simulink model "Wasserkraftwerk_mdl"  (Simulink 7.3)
settings: Solver=ode23tb  StartTime=0.0  StopTime=1000  MaxStep=0.1  RelTol=1e-4
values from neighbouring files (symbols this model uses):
  A_V0 = 0.518    [Parameter_sim.m]
  A_W = 5^2*pi    (= 78.5398163397)    [Parameter_sim.m]
  c_d = 0.9658    [Parameter_sim.m]
  d_F = 2    [Parameter_sim.m]
  d_T = 3    [Parameter_sim.m]
  d_Turb = 5.35    [Parameter_sim.m]
  g = 9.81    [Parameter_sim.m]
  h_R = 413    [Parameter_sim.m]
  h_W0 = 390    [Parameter_sim.m]
  h_W_IC = 413    [Parameter_sim.m]
  I_IC = 0    [Parameter_sim.m]
  kappa = 8.7*10^3    (= 8700)    [Parameter_sim.m]
  l_F = 741    [Parameter_sim.m]
  L_net = 0.1    [Parameter_sim.m]
  l_T = 2000    [Parameter_sim.m]
  L_tot = L_G+L_net    (= 0.2)    [Parameter_sim.m]
  lambda_F = 0.0153    [Parameter_sim.m]
  lambda_T = 0.0182    [Parameter_sim.m]
  lambda_W = 4.0738    [Parameter_sim.m]
  omega_IC = 0    [Parameter_sim.m]
  p_0 = 0    [Parameter_sim.m]
  R_net = 165    [Parameter_sim.m]
  R_tot = R_G+R_net    (= 175)    [Parameter_sim.m]
  rho = 1000    [Parameter_sim.m]
  sigma_0 = 6.2790e-010    (= 6.279e-10)    [Parameter_sim.m]
  Theta = 5.4997*10^3    (= 5499.7)    [Parameter_sim.m]
  v_F_IC = 0    [Parameter_sim.m]
  V_F_IC = l_F*pi*d_F^2/4    (= 2327.92015631)    [Parameter_sim.m]
  v_T_IC = 0    [Parameter_sim.m]
  x_IC = 0    [Parameter_sim.m]
undefined symbols (not defined in the file or in its folder): sigbuilder_block

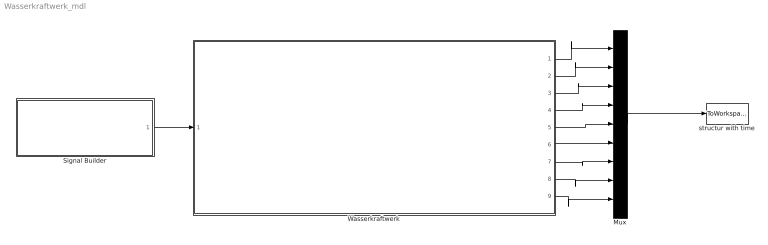
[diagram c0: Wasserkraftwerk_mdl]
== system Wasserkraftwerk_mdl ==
  Mux : Mux  Inputs=9
  Signal Builder : Subsystem  Tag=STV Subsys  LoadFcn=sigbuilder_block('load');  StartFcn=sigbuilder_block('start');  StopFcn=sigbuilder_block('stop');  ClipboardFcn=sigbuilder_block('clipboard');
  Wasserkraftwerk : Subsystem
  structur with time : ToWorkspace  VariableName=sim_daten  SampleTime=-1  SaveFormat=Structure With Time
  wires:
  Signal Builder/1(u) -> Wasserkraftwerk/1(u)
  Mux/1 -> structur with time/1
  Wasserkraftwerk/1(x) -> Mux/1
  Wasserkraftwerk/2(h_W) -> Mux/2
  Wasserkraftwerk/3(p_F) -> Mux/3
  Wasserkraftwerk/4(V_flw_T) -> Mux/4
  Wasserkraftwerk/5(V_flw_F) -> Mux/5
  Wasserkraftwerk/6(omega) -> Mux/6
  Wasserkraftwerk/7(U) -> Mux/7
  Wasserkraftwerk/8(I) -> Mux/8
  Wasserkraftwerk/9(P) -> Mux/9

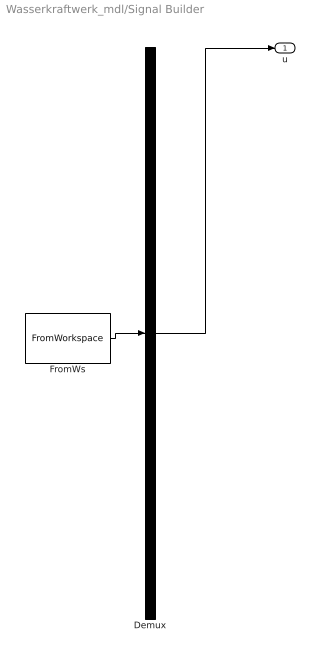
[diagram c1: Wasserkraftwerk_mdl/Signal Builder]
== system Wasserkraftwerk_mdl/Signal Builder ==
  Demux : Demux  Tag=STV Demux  Outputs=1
  FromWs : FromWorkspace  Tag=STV FromWs  VariableName=tuvar  SampleTime=0  SigBuilderData=DataTag0  VnvData=DataTag1
  u : Outport  Tag=STV Outport  OutDataType=sfix(16)  OutScaling=2^0
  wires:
  Demux/1 -> u/1
  FromWs/1 -> Demux/1

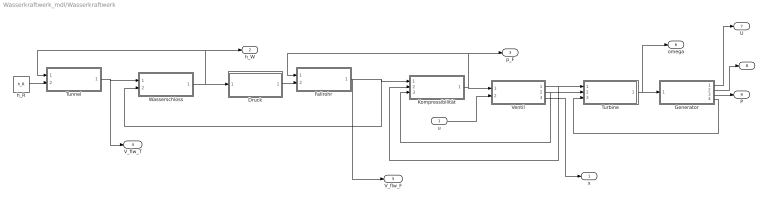
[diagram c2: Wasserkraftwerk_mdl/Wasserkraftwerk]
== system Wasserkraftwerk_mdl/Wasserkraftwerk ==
  u : Inport  OutDataType=sfix(16)  OutScaling=2^0
  Druck : Subsystem
  Fallrohr : Subsystem
  Generator : Subsystem
  Kompressibilität : Subsystem
  Tunnel : Subsystem
  Turbine : Subsystem
  Ventil : Subsystem
  Wasserschloss : Subsystem
  h_R : Constant  Value=h_R  OutDataType=sfix(16)  OutScaling=2^0
  x : Outport  OutDataType=sfix(16)  OutScaling=2^0
  h_W : Outport  Port=2  OutDataType=sfix(16)  OutScaling=2^0
  p_F : Outport  Port=3  OutDataType=sfix(16)  OutScaling=2^0
  V_flw_T : Outport  Port=4  OutDataType=sfix(16)  OutScaling=2^0
  V_flw_F : Outport  Port=5  OutDataType=sfix(16)  OutScaling=2^0
  omega : Outport  Port=6  OutDataType=sfix(16)  OutScaling=2^0
  U : Outport  Port=7  OutDataType=sfix(16)  OutScaling=2^0
  I : Outport  Port=8  OutDataType=sfix(16)  OutScaling=2^0
  P : Outport  Port=9  OutDataType=sfix(16)  OutScaling=2^0
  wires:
  Wasserschloss/1(h_W) -> Druck/1(h_W), Tunnel/1(h_W), h_W/1
  Kompressibilität/1(p_F) -> Ventil/1(p_F), Fallrohr/1(p_F), p_F/1
  Ventil/1(v_V) -> Kompressibilität/2(v_V), Turbine/1(v_V)
  Turbine/1(omega) -> Generator/1(omega), omega/1
  Ventil/2(A_V) -> Kompressibilität/3(A_V), Turbine/2(A_V)
  Generator/1(U) -> U/1
  Generator/2(I) -> I/1
  u/1 -> Ventil/2(u)
  Druck/1(p_W) -> Fallrohr/2(p_W)
  Generator/4(T_G) -> Turbine/3(T_G)
  Ventil/3(x) -> x/1
  Tunnel/1(V_flw_T) -> V_flw_T/1, Wasserschloss/1(V_flw_T)
  Fallrohr/1(V_flw_F) -> Kompressibilität/1(V_flw_F), Wasserschloss/2(V_flw_F), V_flw_F/1
  Generator/3(P) -> P/1
  h_R/1 -> Tunnel/2(h_R)

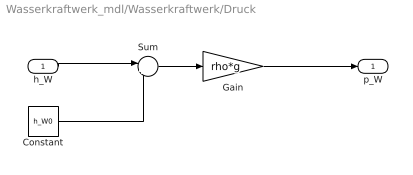
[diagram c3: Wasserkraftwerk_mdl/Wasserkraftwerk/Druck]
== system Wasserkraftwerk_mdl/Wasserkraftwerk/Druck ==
  h_W : Inport  OutDataType=sfix(16)  OutScaling=2^0
  Constant : Constant  Value=h_W0  OutDataType=sfix(16)  OutScaling=2^0
  Gain : Gain  Gain=rho*g  ParameterDataType=sfix(16)  ParameterScaling=2^0  OutDataType=sfix(16)  OutScaling=2^0
  Sum : Sum  Inputs=|+-  OutDataType=sfix(16)  OutScaling=2^0
  p_W : Outport  OutDataType=sfix(16)  OutScaling=2^0
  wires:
  h_W/1 -> Sum/1
  Constant/1 -> Sum/2
  Sum/1 -> Gain/1
  Gain/1 -> p_W/1

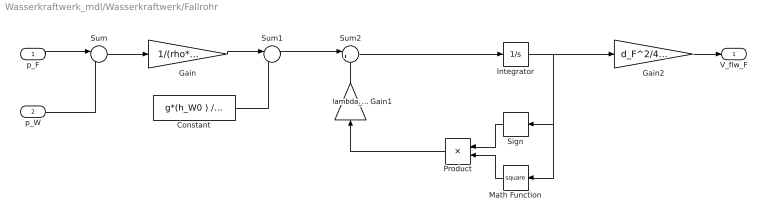
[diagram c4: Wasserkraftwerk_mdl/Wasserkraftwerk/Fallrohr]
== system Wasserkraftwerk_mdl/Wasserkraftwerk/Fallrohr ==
  p_F : Inport  OutDataType=sfix(16)  OutScaling=2^0
  p_W : Inport  Port=2  OutDataType=sfix(16)  OutScaling=2^0
  Constant : Constant  Value=g*(h_W0 ) / l_F  OutDataType=sfix(16)  OutScaling=2^0
  Gain : Gain  Gain=1/(rho*l_F)  ParameterDataType=sfix(16)  ParameterScaling=2^0  OutDataType=sfix(16)  OutScaling=2^0
  Gain1 : Gain  Gain=lambda_F/(2*d_F)  ParameterDataType=sfix(16)  ParameterScaling=2^0  OutDataType=sfix(16)  OutScaling=2^0
  Gain2 : Gain  Gain=d_F^2/4*pi  ParameterDataType=sfix(16)  ParameterScaling=2^0  OutDataType=sfix(16)  OutScaling=2^0
  Integrator : Integrator  InitialCondition=v_F_IC
  Math Function : Math  Operator=square  OutDataType=sfix(16)  OutScaling=2^0
  Product : Product  OutDataType=sfix(16)  OutScaling=2^0
  Sign : Signum
  Sum : Sum  Inputs=|-+  OutDataType=sfix(16)  OutScaling=2^0
  Sum1 : Sum  Inputs=|++  OutDataType=sfix(16)  OutScaling=2^0
  Sum2 : Sum  Inputs=|+-  OutDataType=sfix(16)  OutScaling=2^0
  V_flw_F : Outport  OutDataType=sfix(16)  OutScaling=2^0
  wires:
  p_F/1 -> Sum/1
  p_W/1 -> Sum/2
  Sum/1 -> Gain/1
  Gain/1 -> Sum1/1
  Constant/1 -> Sum1/2
  Sum1/1 -> Sum2/1
  Sum2/1 -> Integrator/1
  Sign/1 -> Product/1
  Math Function/1 -> Product/2
  Product/1 -> Gain1/1
  Gain1/1 -> Sum2/2
  Integrator/1 -> Sign/1, Math Function/1, Gain2/1
  Gain2/1 -> V_flw_F/1

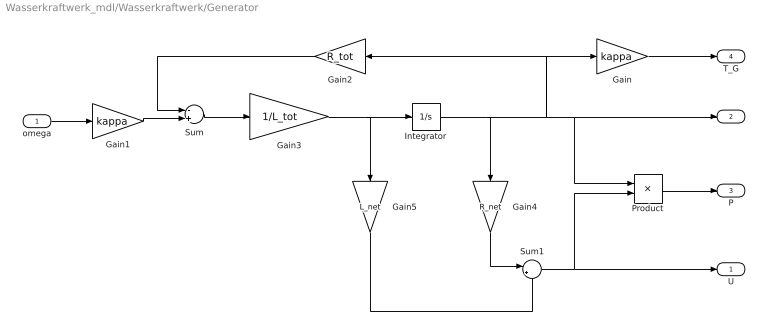
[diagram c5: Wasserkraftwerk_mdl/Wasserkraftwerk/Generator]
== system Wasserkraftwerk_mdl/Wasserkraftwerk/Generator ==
  omega : Inport  OutDataType=sfix(16)  OutScaling=2^0
  Gain : Gain  Gain=kappa  ParameterDataType=sfix(16)  ParameterScaling=2^0  OutDataType=sfix(16)  OutScaling=2^0
  Gain1 : Gain  Gain=kappa  ParameterDataType=sfix(16)  ParameterScaling=2^0  OutDataType=sfix(16)  OutScaling=2^0
  Gain2 : Gain  Gain=R_tot  ParameterDataType=sfix(16)  ParameterScaling=2^0  OutDataType=sfix(16)  OutScaling=2^0
  Gain3 : Gain  Gain=1/L_tot  ParameterDataType=sfix(16)  ParameterScaling=2^0  OutDataType=sfix(16)  OutScaling=2^0
  Gain4 : Gain  Gain=R_net  ParameterDataType=sfix(16)  ParameterScaling=2^0  OutDataType=sfix(16)  OutScaling=2^0
  Gain5 : Gain  Gain=L_net  ParameterDataType=sfix(16)  ParameterScaling=2^0  OutDataType=sfix(16)  OutScaling=2^0
  Integrator : Integrator  InitialCondition=I_IC
  Product : Product  OutDataType=sfix(16)  OutScaling=2^0
  Sum : Sum  Inputs=-+  OutDataType=sfix(16)  OutScaling=2^0
  Sum1 : Sum  Inputs=|++  OutDataType=sfix(16)  OutScaling=2^0
  U : Outport  OutDataType=sfix(16)  OutScaling=2^0
  I : Outport  Port=2  OutDataType=sfix(16)  OutScaling=2^0
  P : Outport  Port=3  OutDataType=sfix(16)  OutScaling=2^0
  T_G : Outport  Port=4  OutDataType=sfix(16)  OutScaling=2^0
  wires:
  Integrator/1 -> Gain/1, Gain2/1, I/1, Product/1, Gain4/1
  Gain/1 -> T_G/1
  omega/1 -> Gain1/1
  Gain2/1 -> Sum/1
  Gain1/1 -> Sum/2
  Sum/1 -> Gain3/1
  Gain3/1 -> Gain5/1, Integrator/1
  Sum1/1 -> U/1, Product/2
  Gain4/1 -> Sum1/1
  Gain5/1 -> Sum1/2
  Product/1 -> P/1

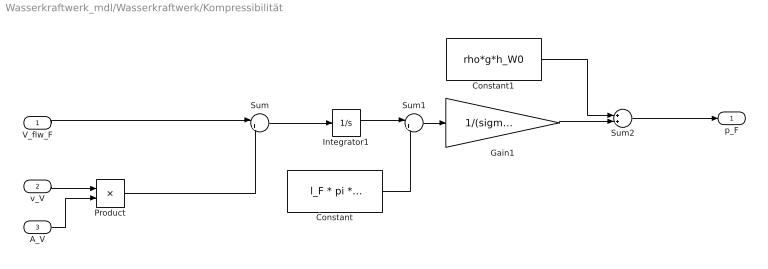
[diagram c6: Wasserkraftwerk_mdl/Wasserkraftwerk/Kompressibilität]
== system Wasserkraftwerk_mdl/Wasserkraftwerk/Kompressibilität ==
  V_flw_F : Inport  OutDataType=sfix(16)  OutScaling=2^0
  v_V : Inport  Port=2  OutDataType=sfix(16)  OutScaling=2^0
  A_V : Inport  Port=3  OutDataType=sfix(16)  OutScaling=2^0
  Constant : Constant  Value=l_F * pi * d_F^2 / 4  OutDataType=sfix(16)  OutScaling=2^0
  Constant1 : Constant  Value=rho*g*h_W0  OutDataType=sfix(16)  OutScaling=2^0
  Gain1 : Gain  Gain=1/(sigma_0 * l_F*pi*d_F^2/4)  ParameterDataType=sfix(16)  ParameterScaling=2^0  OutDataType=sfix(16)  OutScaling=2^0
  Integrator1 : Integrator  InitialCondition=V_F_IC
  Product : Product  OutDataType=sfix(16)  OutScaling=2^0
  Sum : Sum  Inputs=|+-  OutDataType=sfix(16)  OutScaling=2^0
  Sum1 : Sum  Inputs=|+-  OutDataType=sfix(16)  OutScaling=2^0
  Sum2 : Sum  OutDataType=sfix(16)  OutScaling=2^0
  p_F : Outport  OutDataType=sfix(16)  OutScaling=2^0
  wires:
  v_V/1 -> Product/1
  A_V/1 -> Product/2
  Product/1 -> Sum/2
  Sum/1 -> Integrator1/1
  Constant/1 -> Sum1/2
  Sum1/1 -> Gain1/1
  Integrator1/1 -> Sum1/1
  Gain1/1 -> Sum2/2
  Sum2/1 -> p_F/1
  Constant1/1 -> Sum2/1
  V_flw_F/1 -> Sum/1

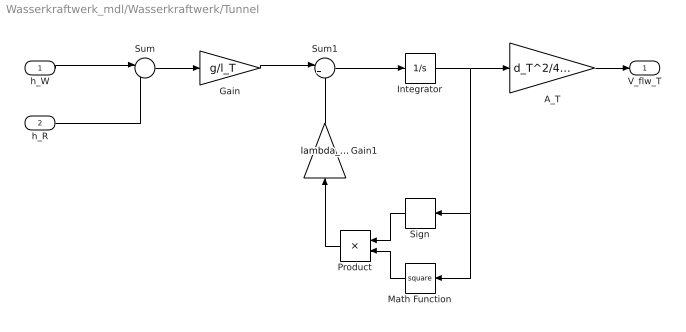
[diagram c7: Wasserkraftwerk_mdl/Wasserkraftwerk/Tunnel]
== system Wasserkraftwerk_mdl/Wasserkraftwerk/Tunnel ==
  h_W : Inport  OutDataType=sfix(16)  OutScaling=2^0
  h_R : Inport  Port=2  OutDataType=sfix(16)  OutScaling=2^0
  A_T : Gain  Gain=d_T^2/4*pi  ParameterDataType=sfix(16)  ParameterScaling=2^0  OutDataType=sfix(16)  OutScaling=2^0
  Gain : Gain  Gain=g/l_T  ParameterDataType=sfix(16)  ParameterScaling=2^0  OutDataType=sfix(16)  OutScaling=2^0
  Gain1 : Gain  Gain=lambda_T/(2*d_T)  ParameterDataType=sfix(16)  ParameterScaling=2^0  OutDataType=sfix(16)  OutScaling=2^0
  Integrator : Integrator  InitialCondition=v_T_IC
  Math Function : Math  Operator=square  OutDataType=sfix(16)  OutScaling=2^0
  Product : Product  OutDataType=sfix(16)  OutScaling=2^0
  Sign : Signum
  Sum : Sum  Inputs=|-+  OutDataType=sfix(16)  OutScaling=2^0
  Sum1 : Sum  Inputs=|+-  OutDataType=sfix(16)  OutScaling=2^0
  V_flw_T : Outport  OutDataType=sfix(16)  OutScaling=2^0
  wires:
  Integrator/1 -> Sign/1, Math Function/1, A_T/1
  h_W/1 -> Sum/1
  Sum/1 -> Gain/1
  Gain/1 -> Sum1/1
  Gain1/1 -> Sum1/2
  Sum1/1 -> Integrator/1
  Product/1 -> Gain1/1
  Sign/1 -> Product/1
  Math Function/1 -> Product/2
  h_R/1 -> Sum/2
  A_T/1 -> V_flw_T/1

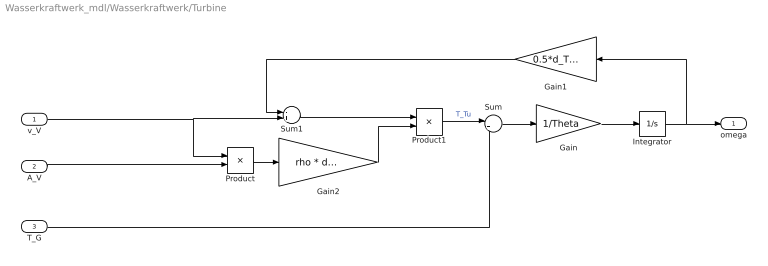
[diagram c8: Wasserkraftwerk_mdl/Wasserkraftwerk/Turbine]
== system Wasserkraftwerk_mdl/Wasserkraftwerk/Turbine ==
  v_V : Inport  OutDataType=sfix(16)  OutScaling=2^0
  A_V : Inport  Port=2  OutDataType=sfix(16)  OutScaling=2^0
  T_G : Inport  Port=3  OutDataType=sfix(16)  OutScaling=2^0
  Gain : Gain  Gain=1/Theta  ParameterDataType=sfix(16)  ParameterScaling=2^0  OutDataType=sfix(16)  OutScaling=2^0
  Gain1 : Gain  Gain=0.5*d_Turb  ParameterDataType=sfix(16)  ParameterScaling=2^0  OutDataType=sfix(16)  OutScaling=2^0
  Gain2 : Gain  Gain=rho * d_Turb  ParameterDataType=sfix(16)  ParameterScaling=2^0  OutDataType=sfix(16)  OutScaling=2^0
  Integrator : Integrator  InitialCondition=omega_IC
  Product : Product  OutDataType=sfix(16)  OutScaling=2^0
  Product1 : Product  OutDataType=sfix(16)  OutScaling=2^0
  Sum : Sum  Inputs=|+-  OutDataType=sfix(16)  OutScaling=2^0
  Sum1 : Sum  Inputs=-+  OutDataType=sfix(16)  OutScaling=2^0
  omega : Outport  OutDataType=sfix(16)  OutScaling=2^0
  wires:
  Integrator/1 -> omega/1, Gain1/1
  Gain/1 -> Integrator/1
  Sum/1 -> Gain/1
  T_G/1 -> Sum/2
  v_V/1 -> Product/1, Sum1/2
  A_V/1 -> Product/2
  Gain1/1 -> Sum1/1
  Product/1 -> Gain2/1
  Sum1/1 -> Product1/1
  Gain2/1 -> Product1/2
  Product1/1 -> Sum/1  "T_Tu"

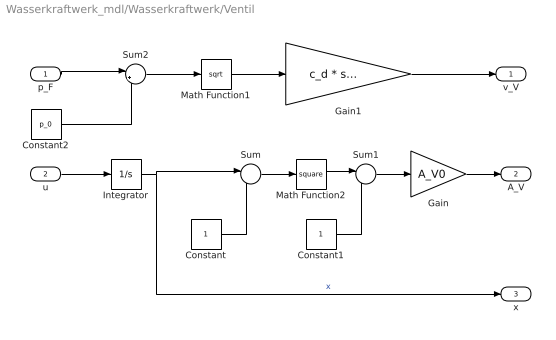
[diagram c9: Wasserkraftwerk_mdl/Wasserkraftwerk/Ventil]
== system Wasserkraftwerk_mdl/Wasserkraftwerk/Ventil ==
  p_F : Inport  OutDataType=sfix(16)  OutScaling=2^0
  u : Inport  Port=2  OutDataType=sfix(16)  OutScaling=2^0
  Constant : Constant  OutDataType=sfix(16)  OutScaling=2^0
  Constant1 : Constant  OutDataType=sfix(16)  OutScaling=2^0
  Constant2 : Constant  Value=p_0  OutDataType=sfix(16)  OutScaling=2^0
  Gain : Gain  Gain=A_V0  ParameterDataType=sfix(16)  ParameterScaling=2^0  OutDataType=sfix(16)  OutScaling=2^0
  Gain1 : Gain  Gain=c_d * sqrt(2/rho)  ParameterDataType=sfix(16)  ParameterScaling=2^0  OutDataType=sfix(16)  OutScaling=2^0
  Integrator : Integrator  InitialCondition=x_IC  LimitOutput=on  UpperSaturationLimit=1  LowerSaturationLimit=0
  Math Function1 : Math  Operator=sqrt  OutDataType=sfix(16)  OutScaling=2^0
  Math Function2 : Math  Operator=square  OutDataType=sfix(16)  OutScaling=2^0
  Sum : Sum  Inputs=|-+  OutDataType=sfix(16)  OutScaling=2^0
  Sum1 : Sum  Inputs=|-+  OutDataType=sfix(16)  OutScaling=2^0
  Sum2 : Sum  Inputs=|+-  OutDataType=sfix(16)  OutScaling=2^0
  v_V : Outport  OutDataType=sfix(16)  OutScaling=2^0
  A_V : Outport  Port=2  OutDataType=sfix(16)  OutScaling=2^0
  x : Outport  Port=3  OutDataType=sfix(16)  OutScaling=2^0
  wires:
  u/1 -> Integrator/1
  Integrator/1 -> Sum/1, x/1  "x"
  Constant/1 -> Sum/2
  Sum/1 -> Math Function2/1
  Constant1/1 -> Sum1/2
  Sum1/1 -> Gain/1
  p_F/1 -> Sum2/1
  Constant2/1 -> Sum2/2
  Sum2/1 -> Math Function1/1
  Math Function1/1 -> Gain1/1
  Gain1/1 -> v_V/1
  Math Function2/1 -> Sum1/1
  Gain/1 -> A_V/1

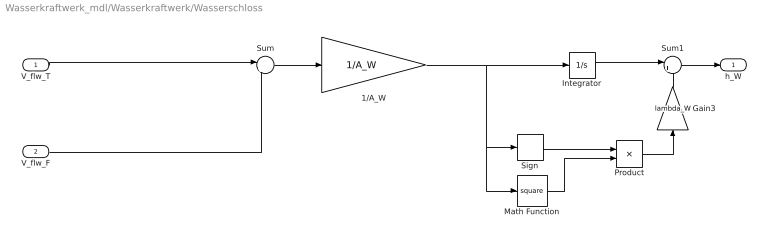
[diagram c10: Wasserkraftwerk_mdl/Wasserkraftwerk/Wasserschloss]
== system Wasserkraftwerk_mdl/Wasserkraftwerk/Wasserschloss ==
  V_flw_T : Inport  OutDataType=sfix(16)  OutScaling=2^0
  V_flw_F : Inport  Port=2  OutDataType=sfix(16)  OutScaling=2^0
  1/A_W : Gain  Gain=1/A_W  ParameterDataType=sfix(16)  ParameterScaling=2^0  OutDataType=sfix(16)  OutScaling=2^0
  Gain3 : Gain  Gain=lambda_W  ParameterDataType=sfix(16)  ParameterScaling=2^0  OutDataType=sfix(16)  OutScaling=2^0
  Integrator : Integrator  InitialCondition=h_W_IC
  Math Function : Math  Operator=square  OutDataType=sfix(16)  OutScaling=2^0
  Product : Product  OutDataType=sfix(16)  OutScaling=2^0
  Sign : Signum
  Sum : Sum  Inputs=|+-  OutDataType=sfix(16)  OutScaling=2^0
  Sum1 : Sum  Inputs=|++  OutDataType=sfix(16)  OutScaling=2^0
  h_W : Outport  OutDataType=sfix(16)  OutScaling=2^0
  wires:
  V_flw_F/1 -> Sum/2
  V_flw_T/1 -> Sum/1
  Sum/1 -> 1/A_W/1
  1/A_W/1 -> Sign/1, Math Function/1, Integrator/1
  Sign/1 -> Product/1
  Math Function/1 -> Product/2
  Product/1 -> Gain3/1
  Gain3/1 -> Sum1/2
  Sum1/1 -> h_W/1
  Integrator/1 -> Sum1/1
